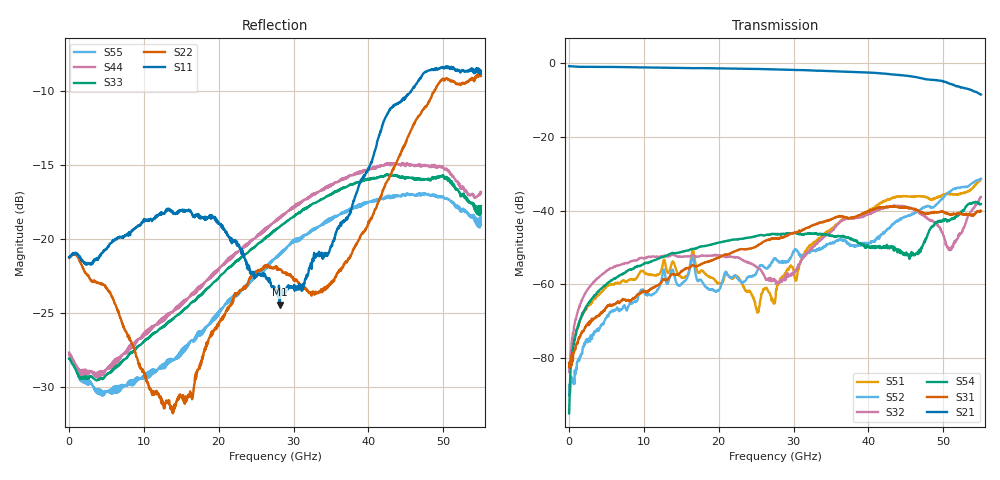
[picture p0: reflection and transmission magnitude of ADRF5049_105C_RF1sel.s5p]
! Device  : ADRF5049
! Description: Silicon SP4T Switch Non-Reflective
! Frequency:  9kHz -  45 GHz
! Ports:
!  RFC = Port 1
!  RF1 = Port 2
!  RF2 = Port 3
!	 RF3 = Port 4
!  RF4 = Port 5
! VSS  =  +3.30 Volts
! VDD  =  -3.30 Volts
! EN  =  0.00 Volts
! LS  =  0.00 Volts
! V1  =  0.00 Volts
! V2  =  0.00 Volts
! Data:  Data was collected using an calibrated 4 port network analyzer.
! Notes: Analog Devices supplies this data as a sample of measured data
!  for this product.  Your particular data for this product may vary.
!  Data was taken at 105C degrees C.
!  Analog Devices reserves the right to change this data at anytime.
# hz S db R 50
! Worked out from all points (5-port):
!   1100 points, 50 MHz to 55 GHz, reference 50 ohm
!   strongest paths, dB at 50 MHz, 13.8 GHz, 27.55 GHz, 41.3 GHz, 55 GHz:
!     S21: -0.9, -1.3, -1.8, -2.8, -8.6
!     S31: -81.3, -57.2, -47.6, -39.3, -40.1
!     S54: -95.0, -51.5, -46.4, -49.7, -38.2
!     S32: -83.8, -52.0, -58.8, -39.8, -36.3
!     S52: -87.3, -56.0, -53.1, -47.1, -31.4
!     S51: -81.4, -54.0, -64.4, -38.4, -31.5
!   lowest |S11| = -24.5 dB at 28.15 GHz (marker M1), VSWR 1.13, Z = 53.1 - j5.35 ohm
!   |S11| at or under -10 dB: start of sweep to 45.67 GHz
